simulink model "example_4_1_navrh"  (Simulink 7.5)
settings: Solver=ode45  StartTime=0.0  StopTime=2  RelTol=1e-3
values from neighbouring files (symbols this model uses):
  A = [dh1_h10 dh1_h20 0    [podklad.m]    (also in testx.m = [ -0.195 0.195; 0.195 -0.205]; kockaLQG.m = [0 1 0 0 0; kockaLQR.m = [0 1 0 0 0; kulicka_na_tyci_LQG_podklad.m = [0 0;1 0])
  B = [dh1_q0    [podklad.m]    (also in testx.m = [0.0047; 0]; kockaLQG.m = [0; kockaLQR.m = [0; kulicka_na_tyci_LQG_podklad.m = [7.14;0])
  C = [0 0 1]    [podklad.m]    (also in testx.m = [0 1]; kockaLQG.m = [1 0 0 0 0]; kockaLQR.m = [1 0 0 0 0]; kulicka_na_tyci_LQG_podklad.m = [0 1])
  D = 0    [podklad.m]    (also in testx.m = [0]; kockaLQG.m = [0]; kockaLQR.m = [0]; kulicka_na_tyci_LQG_podklad.m)
  g = 9.81    [podklad.m]    (also in kockaLQG.m; kockaLQR.m; nadrze_soustava.m; nadoby.m)
  kc = kf/(ki^2)    (= 5.56473829201e-06)    [podklad.m]
  Kfv = 0.02    [podklad.m]
  ki = 0.33    [podklad.m]
  Kreg3 = lqg(sys,0.0001*eye(4),QMV,10000)    [podklad.m]
  mk = 8.37e-3    (= 0.00837)    [podklad.m]    (also in kockaLQG.m = 1; kockaLQR.m = 1)
  Ta = 3e-3    (= 0.003)    [podklad.m]
  x0 = 8.26e-3    (= 0.00826)    [podklad.m]
undefined symbols (not defined in the file or in its folder): float
libraries: simulink x1

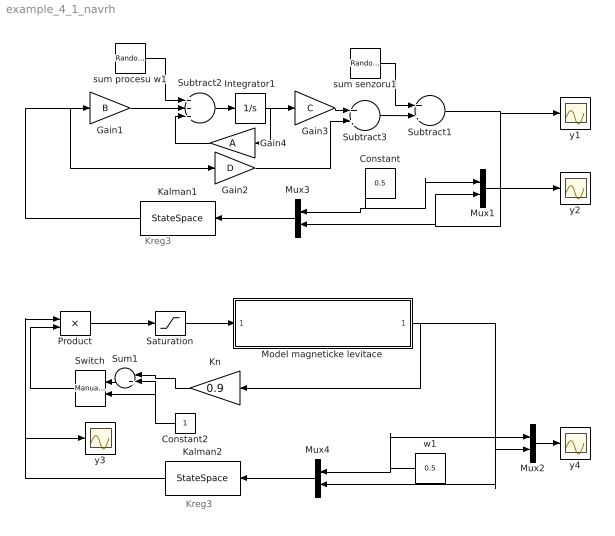
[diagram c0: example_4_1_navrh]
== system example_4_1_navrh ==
  note: Kreg3
  note: Kreg3
  Constant : Constant  Value=0.5  OutDataType=sfix(16)  OutScaling=2^0
  Constant2 : Constant  OutDataType=sfix(16)  OutScaling=2^0
  Gain1 : Gain  Gain=B  Multiplication=Matrix(K*u)  ParameterDataType=sfix(16)  ParameterScaling=2^0  OutDataType=sfix(16)  OutScaling=2^0
  Gain2 : Gain  Gain=D  Multiplication=Matrix(K*u)  ParameterDataType=sfix(16)  ParameterScaling=2^0  OutDataType=sfix(16)  OutScaling=2^0
  Gain3 : Gain  Gain=C  Multiplication=Matrix(K*u)  ParameterDataType=sfix(16)  ParameterScaling=2^0  OutDataType=sfix(16)  OutScaling=2^0
  Gain4 : Gain  Gain=A  Multiplication=Matrix(K*u)  ParameterDataType=sfix(16)  ParameterScaling=2^0  OutDataType=sfix(16)  OutScaling=2^0
  Integrator1 : Integrator  InitialCondition=0.5
  Kalman1 : StateSpace  A=Kreg3.a  B=Kreg3.b  C=Kreg3.c  D=Kreg3.d
  Kalman2 : StateSpace  A=Kreg3.a  B=Kreg3.b  C=Kreg3.c  D=Kreg3.d
  Kn : Gain  Gain=0.9  ParameterDataType=sfix(16)  ParameterScaling=2^0  OutDataType=sfix(16)  OutScaling=2^0
  Model magneticke levitace : Subsystem
  Mux{1..4} (4 alike) : Mux  Inputs=2
  Product : Product  OutDataType=sfix(16)  OutScaling=2^0
  Saturation : Saturate  UpperLimit=1  LowerLimit=0
  Subtract1 : Sum  OutDataType=sfix(16)  OutScaling=2^-10
  Subtract2 : Sum  Inputs=+++  OutDataType=sfix(16)  OutScaling=2^-10
  Subtract3 : Sum  OutDataType=sfix(16)  OutScaling=2^-10
  Sum1 : Sum  Inputs=-+  OutDataType=sfix(16)  OutScaling=2^0
  Switch : simulink/Signal Routing/Manual Switch  SystemSampleTime=-1  sw=1  action=0  varsize=off
  sum procesu w1 : RandomNumber  Variance=0.0001  SampleTime=0
  sum senzoru1 : RandomNumber  Variance=0.000001  SampleTime=0
  w1 : Constant  Value=0.5  OutDataType=sfix(16)  OutScaling=2^0
  y{1..4} (4 alike) : Scope
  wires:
  Integrator1/1 -> Gain4/1, Gain3/1
  Subtract2/1 -> Integrator1/1
  Subtract3/1 -> Subtract1/2
  Subtract1/1 -> y1/1, Mux3/2, Mux1/2
  Gain3/1 -> Subtract3/1
  Gain2/1 -> Subtract3/2
  Gain4/1 -> Subtract2/3
  Gain1/1 -> Subtract2/2
  sum procesu w1/1 -> Subtract2/1
  sum senzoru1/1 -> Subtract1/1
  Kalman1/1 -> Gain1/1, Gain2/1
  Mux3/1 -> Kalman1/1
  Constant/1 -> Mux3/1, Mux1/1
  Mux1/1 -> y2/1
  Mux4/1 -> Kalman2/1
  Mux2/1 -> y4/1
  Kalman2/1 -> Product/1, y3/1
  Model magneticke levitace/1(y - output voltage) -> Kn/1, Mux4/2, Mux2/2
  Product/1 -> Saturation/1
  Kn/1 -> Sum1/1
  Constant2/1 -> Sum1/2, Switch/2
  Saturation/1 -> Model magneticke levitace/1(u - Input voltage [MU])
  Sum1/1 -> Switch/1
  Switch/1 -> Product/2
  w1/1 -> Mux4/1, Mux2/1

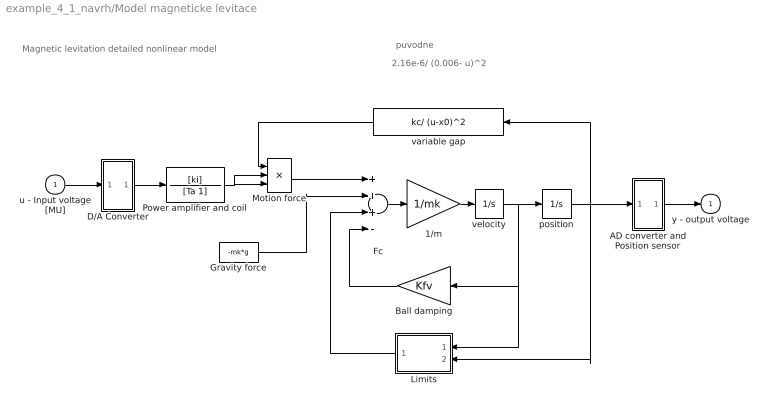
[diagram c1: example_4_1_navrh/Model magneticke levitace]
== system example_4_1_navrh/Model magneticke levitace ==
  note: Magnetic levitation detailed nonlinear model
  note: puvodne
  note: 2.16e-6/ (0.006- u)^2
  u - Input voltage [MU] : Inport  OutDataType=sfix(16)  OutScaling=2^0
  1/m : Gain  Gain=1/mk  ParameterDataType=sfix(16)  ParameterScaling=2^0  OutDataType=sfix(16)  OutScaling=2^0
  AD converter and Position sensor : Subsystem
  Ball damping : Gain  Gain=Kfv  ParameterDataType=sfix(16)  ParameterScaling=2^0  OutDataType=sfix(16)  OutScaling=2^0
  D/A Converter : Subsystem
  Fc : Sum  Inputs=+++-  OutDataType=sfix(16)  OutScaling=2^0
  Gravity force : Constant  Value=-mk*g  OutDataType=sfix(16)  OutScaling=2^0
  Limits : Subsystem
  Motion force : Product  Inputs=3  OutDataType=sfix(16)  OutScaling=2^0
  Power amplifier and coil : TransferFcn  Numerator=[ki]  Denominator=[Ta 1]
  position : Integrator  LimitOutput=on  UpperSaturationLimit=0.0063  LowerSaturationLimit=0
  variable gap : Fcn  Expr=kc/ (u-x0)^2
  velocity : Integrator
  y - output voltage : Outport
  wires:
  Power amplifier and coil/1 -> Motion force/2, Motion force/3
  Limits/1(force) -> Fc/3
  position/1 -> AD converter and Position sensor/1(in_1), variable gap/1, Limits/2(position)
  AD converter and Position sensor/1(out_1) -> y - output voltage/1
  u - Input voltage [MU]/1 -> D/A Converter/1(in_1)
  D/A Converter/1(out_1) -> Power amplifier and coil/1
  Gravity force/1 -> Fc/2
  Motion force/1 -> Fc/1
  Fc/1 -> 1/m/1
  1/m/1 -> velocity/1
  variable gap/1 -> Motion force/1
  Ball damping/1 -> Fc/4
  velocity/1 -> position/1, Limits/1(velocity), Ball damping/1

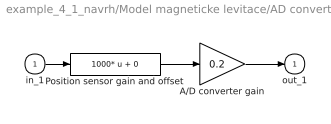
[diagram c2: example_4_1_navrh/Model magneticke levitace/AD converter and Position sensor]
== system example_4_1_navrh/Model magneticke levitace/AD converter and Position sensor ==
  in_1 : Inport  OutDataType=sfix(16)  OutScaling=2^0
  A/D converter gain : Gain  Gain=0.2  ParameterDataType=sfix(16)  ParameterScaling=2^0  OutDataType=sfix(16)  OutScaling=2^0
  Position sensor gain and offset : Fcn  Expr=1000* u + 0
  out_1 : Outport
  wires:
  A/D converter gain/1 -> out_1/1
  Position sensor gain and offset/1 -> A/D converter gain/1
  in_1/1 -> Position sensor gain and offset/1

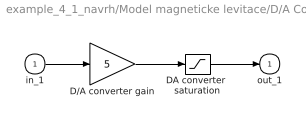
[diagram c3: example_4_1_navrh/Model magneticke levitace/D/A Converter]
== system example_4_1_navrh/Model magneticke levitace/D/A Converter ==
  in_1 : Inport  OutDataType=sfix(16)  OutScaling=2^0
  D/A converter gain : Gain  Gain=5  ParameterDataType=sfix(16)  ParameterScaling=2^0  OutDataType=sfix(16)  OutScaling=2^0
  DA converter  saturation : Saturate  UpperLimit=5  LowerLimit=-5
  out_1 : Outport
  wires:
  D/A converter gain/1 -> DA converter  saturation/1
  DA converter  saturation/1 -> out_1/1
  in_1/1 -> D/A converter gain/1

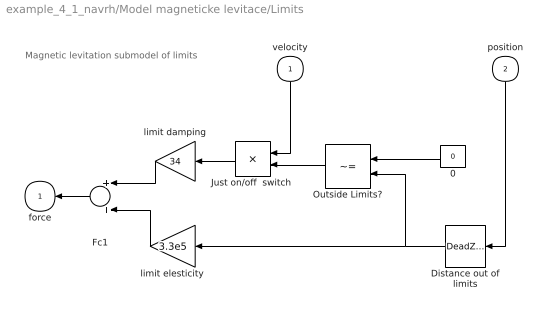
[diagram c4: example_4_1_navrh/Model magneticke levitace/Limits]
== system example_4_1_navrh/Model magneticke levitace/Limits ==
  note: Magnetic levitation submodel of limits
  velocity : Inport  OutDataType=sfix(16)  OutScaling=2^0
  position : Inport  Port=2  OutDataType=sfix(16)  OutScaling=2^0
  0 : Constant  Value=0  OutDataType=sfix(16)  OutScaling=2^0
  Distance out of limits : DeadZone  LowerValue=0  UpperValue=0.0063
  Fc1 : Sum  OutDataType=sfix(16)  OutScaling=2^0
  "Just on/off  switch " : Product  OutDataType=sfix(16)  OutScaling=2^0
  Outside Limits? : RelationalOperator  Operator=~=  LogicOutDataTypeMode=Specify via dialog  LogicDataType=float('double')  OutDataTypeStr=float('double')
  limit damping : Gain  Gain=34  ParameterDataType=sfix(16)  ParameterScaling=2^0  OutDataType=sfix(16)  OutScaling=2^0
  limit elesticity : Gain  Gain=3.3e5  ParameterDataType=sfix(16)  ParameterScaling=2^0  OutDataType=sfix(16)  OutScaling=2^0
  force : Outport
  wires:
  position/1 -> Distance out of limits/1
  Fc1/1 -> force/1
  velocity/1 -> "Just on/off  switch "/1
  "Just on/off  switch "/1 -> limit damping/1
  0/1 -> Outside Limits?/1
  Outside Limits?/1 -> "Just on/off  switch "/2
  limit elesticity/1 -> Fc1/2
  limit damping/1 -> Fc1/1
  Distance out of limits/1 -> limit elesticity/1, Outside Limits?/2
